FUNCTION "ROBOT_INRFACE1" : VOID
TITLE =ROBOT INTERFACE FOR CYCLE OF JOB 0, 1, 2, 3.
AUTHOR : Esposito
FAMILY : EGAL_srl
NAME : ROB_INT1
VERSION : 0.1

BEGIN
NETWORK
TITLE =DEFINITION OF THE CYCLE OF JOB "ZERO" ROBOT 1 AND 2
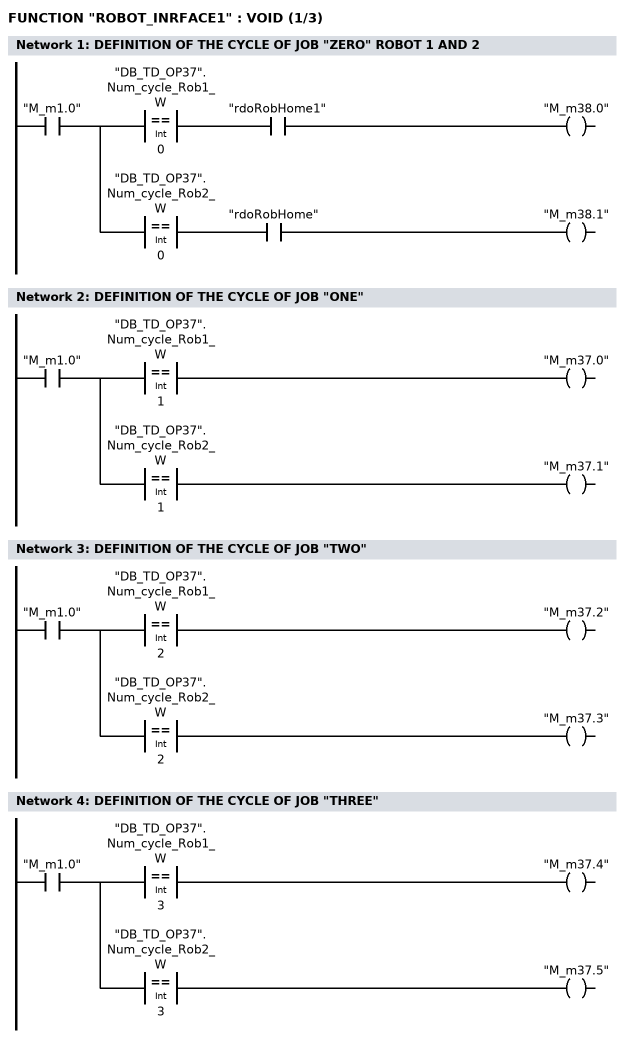
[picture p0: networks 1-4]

      U     "M_m1.0";
      =     L      0.0;
      U     L      0.0;
      U(    ;
      L     "DB_TD_OP37".Num_cycle_Rob1_W;
      L     0;
      ==I   ;
      )     ;
      U     "rdoRobHome1";
      =     "M_m38.0";
      U     L      0.0;
      U(    ;
      L     "DB_TD_OP37".Num_cycle_Rob2_W;
      L     0;
      ==I   ;
      )     ;
      U     "rdoRobHome";
      =     "M_m38.1";
NETWORK
TITLE =DEFINITION OF THE CYCLE OF JOB "ONE"

      U     "M_m1.0";
      =     L      0.0;
      U     L      0.0;
      U(    ;
      L     "DB_TD_OP37".Num_cycle_Rob1_W;
      L     1;
      ==I   ;
      )     ;
      =     "M_m37.0";
      U     L      0.0;
      U(    ;
      L     "DB_TD_OP37".Num_cycle_Rob2_W;
      L     1;
      ==I   ;
      )     ;
      =     "M_m37.1";
NETWORK
TITLE =DEFINITION OF THE CYCLE OF JOB "TWO"

      U     "M_m1.0";
      =     L      0.0;
      U     L      0.0;
      U(    ;
      L     "DB_TD_OP37".Num_cycle_Rob1_W;
      L     2;
      ==I   ;
      )     ;
      =     "M_m37.2";
      U     L      0.0;
      U(    ;
      L     "DB_TD_OP37".Num_cycle_Rob2_W;
      L     2;
      ==I   ;
      )     ;
      =     "M_m37.3";
NETWORK
TITLE =DEFINITION OF THE CYCLE OF JOB "THREE"

      U     "M_m1.0";
      =     L      0.0;
      U     L      0.0;
      U(    ;
      L     "DB_TD_OP37".Num_cycle_Rob1_W;
      L     3;
      ==I   ;
      )     ;
      =     "M_m37.4";
      U     L      0.0;
      U(    ;
      L     "DB_TD_OP37".Num_cycle_Rob2_W;
      L     3;
      ==I   ;
      )     ;
      =     "M_m37.5";
NETWORK
TITLE =CONTROL CAMS ROBOT 1 AND 2 SICUREZZA ROBOT IN PRESSA
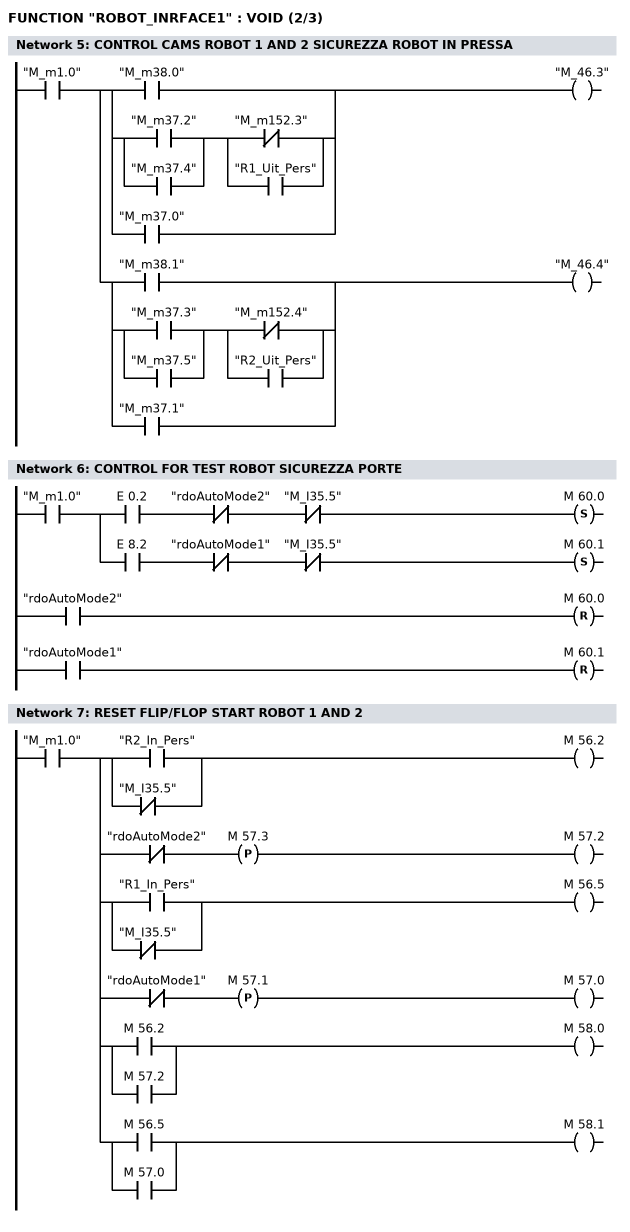
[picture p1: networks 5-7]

      U     "M_m1.0";
      =     L      0.0;
      U     L      0.0;
      U(    ;
      O     "M_m38.0";
      O     ;
      U(    ;
      O     "M_m37.2";
      O     "M_m37.4";
      )     ;
      U(    ;
      ON    "M_m152.3";
      O     "R1_Uit_Pers";
      )     ;
      O     "M_m37.0";
      )     ;
      =     "M_46.3";
      U     L      0.0;
      U(    ;
      O     "M_m38.1";
      O     ;
      U(    ;
      O     "M_m37.3";
      O     "M_m37.5";
      )     ;
      U(    ;
      ON    "M_m152.4";
      O     "R2_Uit_Pers";
      )     ;
      O     "M_m37.1";
      )     ;
      =     "M_46.4";
NETWORK
TITLE =CONTROL FOR TEST ROBOT SICUREZZA PORTE

      U     "M_m1.0";
      =     L      0.0;
      U     L      0.0;
      U     E      0.2;
      UN    "rdoAutoMode2";
      UN    "M_I35.5";
      S     M     60.0;
      U     "rdoAutoMode2";
      R     M     60.0;
      NOP   0;
      U     L      0.0;
      U     E      8.2;
      UN    "rdoAutoMode1";
      UN    "M_I35.5";
      S     M     60.1;
      U     "rdoAutoMode1";
      R     M     60.1;
      NOP   0;
NETWORK
TITLE =RESET FLIP/FLOP START ROBOT 1 AND 2

      U     "M_m1.0";
      =     L      0.0;
      U     L      0.0;
      U(    ;
      O     "R2_In_Pers";
      ON    "M_I35.5";
      )     ;
      =     M     56.2;
      U     L      0.0;
      UN    "rdoAutoMode2";
      FP    M     57.3;
      =     M     57.2;
      U     L      0.0;
      U(    ;
      O     "R1_In_Pers";
      ON    "M_I35.5";
      )     ;
      =     M     56.5;
      U     L      0.0;
      UN    "rdoAutoMode1";
      FP    M     57.1;
      =     M     57.0;
      U     L      0.0;
      U(    ;
      O     M     56.2;
      O     M     57.2;
      )     ;
      =     M     58.0;
      U     L      0.0;
      U(    ;
      O     M     56.5;
      O     M     57.0;
      )     ;
      =     M     58.1;
NETWORK
TITLE =START ROBOT 1 AND 2
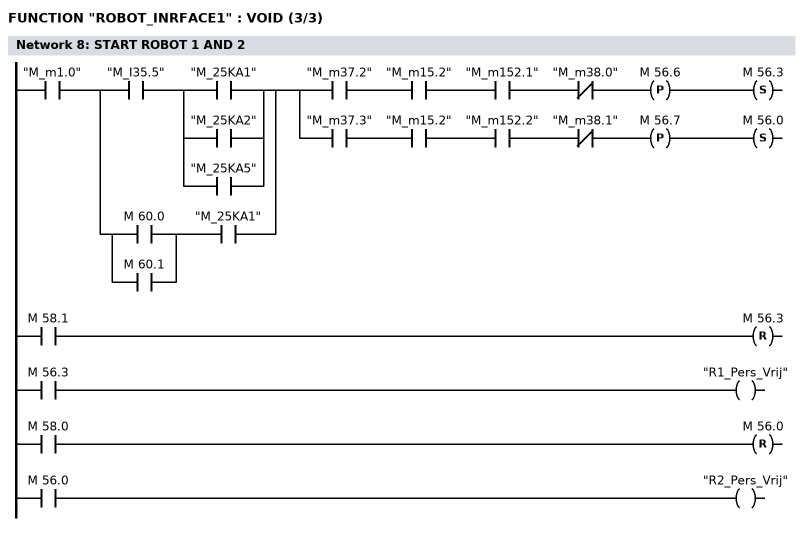
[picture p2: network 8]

      U     "M_m1.0";
      U(    ;
      U     "M_I35.5";
      U(    ;
      O     "M_25KA1";
      O     "M_25KA2";
      O     "M_25KA5";
      )     ;
      O     ;
      U(    ;
      O     M     60.0;
      O     M     60.1;
      )     ;
      U     "M_25KA1";
      )     ;
      =     L      0.0;
      U     L      0.0;
      U     "M_m37.2";
      U     "M_m15.2";
      U     "M_m152.1";
      UN    "M_m38.0";
      FP    M     56.6;
      S     M     56.3;
      U     M     58.1;
      R     M     56.3;
      U     M     56.3;
      =     "R1_Pers_Vrij";
      U     L      0.0;
      U     "M_m37.3";
      U     "M_m15.2";
      U     "M_m152.2";
      UN    "M_m38.1";
      FP    M     56.7;
      S     M     56.0;
      U     M     58.0;
      R     M     56.0;
      U     M     56.0;
      =     "R2_Pers_Vrij";
END_FUNCTION

